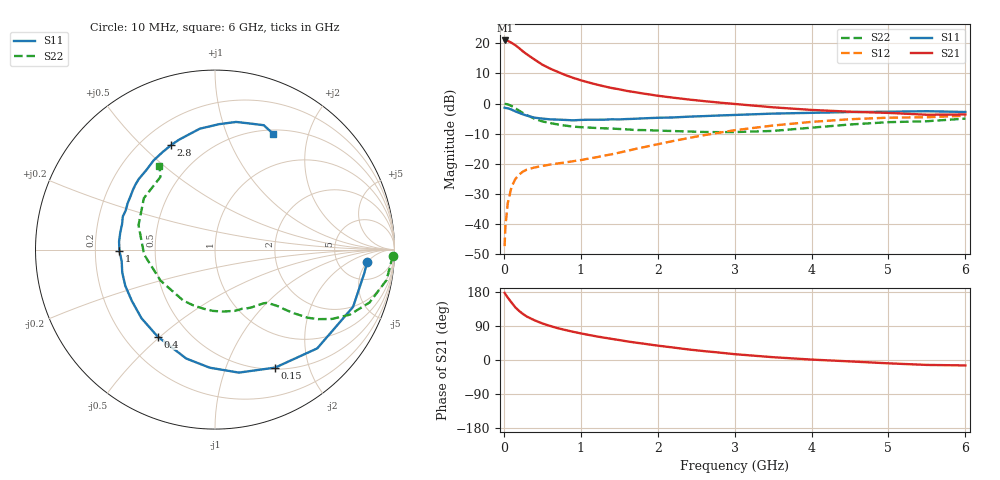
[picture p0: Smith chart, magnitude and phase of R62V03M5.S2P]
! SIEMENS Small Signal Semiconductors
! BFR193
! Si NPN RF Bipolar Junction Transistor in SOT23
! VCE = 2 V  IC = 3.5 mA
! Common Emitter S-Parameters:  May  1996
# GHz  S  MA  R  50
!  f  S11  S21  S12  S22
! GHz  MAG  ANG  MAG  ANG  MAG  ANG  MAG  ANG
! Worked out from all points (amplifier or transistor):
!   36 points, 10 MHz to 6 GHz, reference 50 ohm
!   highest |S21| = 21.0 dB at 20 MHz (marker M1)
!   |S21| within 3 dB of that: start of sweep to 219 MHz
!   unconditionally stable (mu >= 1): 976.1 MHz to 2.024 GHz
!   at 250 MHz: K = 0.34, MSG = 20.0 dB, |S12| = -22.7 dB
!   at 1.4 GHz: K = 1.08, MAG = 9.3 dB, |S12| = -16.9 dB
!   at 6 GHz: K = 0.98, MSG = 0.2 dB, |S12| = -4.1 dB
!   S11 on the Smith chart (normalised r, x): 10 MHz: 10, -5; 150 MHz: 0.52, -1.50; 400 MHz: 0.34, -0.49; 1 GHz: 0.30, -0.01; 2.8 GHz: 0.32, +0.62; 6 GHz: 0.55, +1.48
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0.01  0.8503 -4.8  11.11 177.2  0.0042 89.1  0.9942 -2.0
0.02  0.8419 -9.1  11.23 173.8  0.0088 86.4  0.984 -4.0
0.05  0.8329 -22.5  11.12 165.0  0.0216 78.6  0.9705 -10.1
0.1  0.7921 -44.0  10.26 151.6  0.0409 68.6  0.91 -18.9
0.15  0.7379 -63.0  9.355 138.8  0.0554 59.5  0.8336 -25.8
0.2  0.6982 -79.0  8.339 129.3  0.0657 53.5  0.7571 -30.7
0.25  0.6588 -92.5  7.355 121.2  0.0736 48.7  0.6928 -34.0
0.3  0.6277 -104.8  6.597 114.6  0.0794 45.8  0.6415 -36.3
0.4  0.5805 -123.4  5.39 104.6  0.086 42.4  0.5566 -39.2
0.5  0.5603 -137.0  4.441 96.5  0.0911 41.0  0.5036 -40.9
0.6  0.5443 -148.4  3.82 89.9  0.096 41.1  0.4729 -41.9
0.7  0.539 -158.0  3.367 84.0  0.1003 41.8  0.4481 -43.3
0.8  0.5325 -166.0  2.98 79.1  0.1043 43.4  0.4284 -44.6
1  0.5327 -179.3  2.439 70.2  0.1141 47.5  0.4037 -47.8
1.1  0.5364 175.1  2.245 66.3  0.1207 49.3  0.3973 -50.0
1.6  0.5509 152.1  1.62 49.2  0.1621 56.5  0.3707 -62.6
2.2  0.5854 130.8  1.251 33.0  0.237 57.8  0.3477 -83.2
2.8  0.6316 112.8  1.036 19.6  0.3268 52.4  0.3334 -111.3
3.5  0.6788 97.2  0.864 7.4  0.4297 41.0  0.3491 -150.2
4.5  0.7209 80.6  0.73 -3.7  0.5471 22.9  0.4472 162.3
5.5  0.7444 68.6  0.65 -13.0  0.5904 5.1  0.5062 126.9
6  0.7223 63.3  0.657 -14.3  0.6255 0.0  0.5607 123.5
